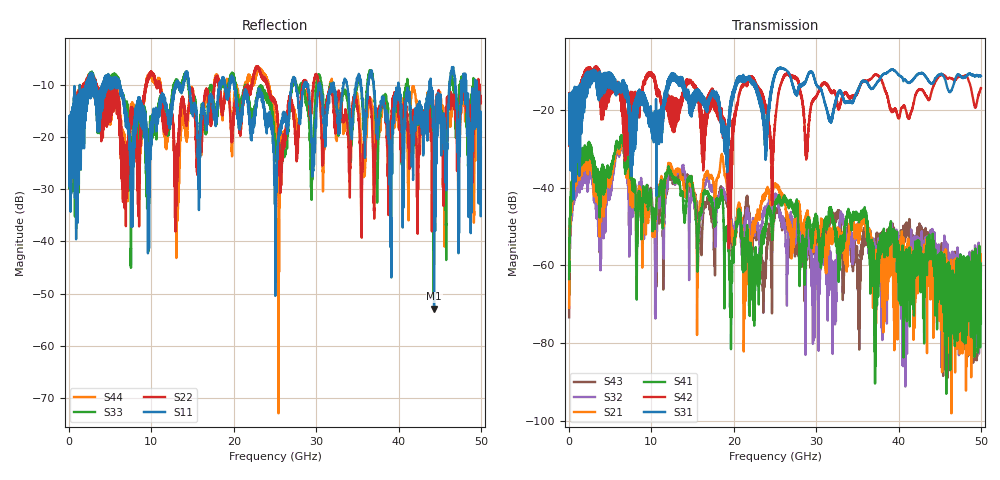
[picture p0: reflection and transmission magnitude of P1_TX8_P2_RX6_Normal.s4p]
!Keysight Technologies,N5225B,MY57041031,A.13.20.10
!Date: Friday, May 31, 2019 11:37:22
!Correction: S11(Full 4 Port(1,2,3,4))
!S12(Full 4 Port(1,2,3,4))
!S13(Full 4 Port(1,2,3,4))
!S14(Full 4 Port(1,2,3,4))
!S21(Full 4 Port(1,2,3,4))
!S22(Full 4 Port(1,2,3,4))
!S23(Full 4 Port(1,2,3,4))
!S24(Full 4 Port(1,2,3,4))
!S31(Full 4 Port(1,2,3,4))
!S32(Full 4 Port(1,2,3,4))
!S33(Full 4 Port(1,2,3,4))
!S34(Full 4 Port(1,2,3,4))
!S41(Full 4 Port(1,2,3,4))
!S42(Full 4 Port(1,2,3,4))
!S43(Full 4 Port(1,2,3,4))
!S44(Full 4 Port(1,2,3,4))
!S4P File: Measurements: <S11,S12,S13,S14>,
!<S21,S22,S23,S24>,
!<S31,S32,S33,S34>,
!<S41,S42,S43,S44>:
# Hz S  dB  R 50.0
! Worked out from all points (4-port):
!   5000 points, 10 MHz to 50 GHz, reference 50 ohm
!   strongest paths, dB at 10 MHz, 12.51 GHz, 25.01 GHz, 37.51 GHz, 50 GHz:
!     S31: -19.5, -10.7, -11.1, -12.7, -11.2
!     S42: -19.5, -16.8, -23.7, -11.2, -14.5
!     S41: -63.5, -36.7, -44.3, -64.9, -74.9
!     S21: -70.9, -35.0, -39.1, -62.9, -66.5
!     S32: -59.4, -35.5, -41.9, -54.8, -61.2
!     S43: -73.4, -37.5, -46.4, -55.0, -59.4
!   lowest |S11| = -52.9 dB at 44.32 GHz (marker M1), VSWR 1.00, Z = 49.8 - j0.149 ohm
!   |S11| at or under -10 dB: 6.184 GHz to 12.93 GHz (6.744 GHz wide, 70.6 % of centre); 20.09 GHz to 26.99 GHz (6.894 GHz wide, 29.3 % of centre); 40 GHz to 43.77 GHz (3.77 GHz wide, 9 % of centre)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
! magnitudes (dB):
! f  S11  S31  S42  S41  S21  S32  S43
! 10 MHz  -19.3  -19.5  -19.5  -63.5  -70.9  -59.4  -73.4
! 960 MHz  -20.3  -21.1  -18.1  -31.2  -33.4  -35.7  -33.4
! 6.4 GHz  -12.1  -14.0  -17.4  -26.6  -27.3  -27.6  -26.9
! 10.39 GHz  -15.9  -25.8  -11.7  -50.1  -51.6  -51.2  -48.6
! 19.68 GHz  -9.2  -17.7  -29.3  -68.2  -50.3  -47.9  -52.1
! 44.32 GHz  -52.9  -12.6  -13.5  -56.4  -61.1  -56.8  -60.0
! 50 GHz  -22.0  -11.2  -14.5  -74.9  -66.5  -61.2  -59.4
